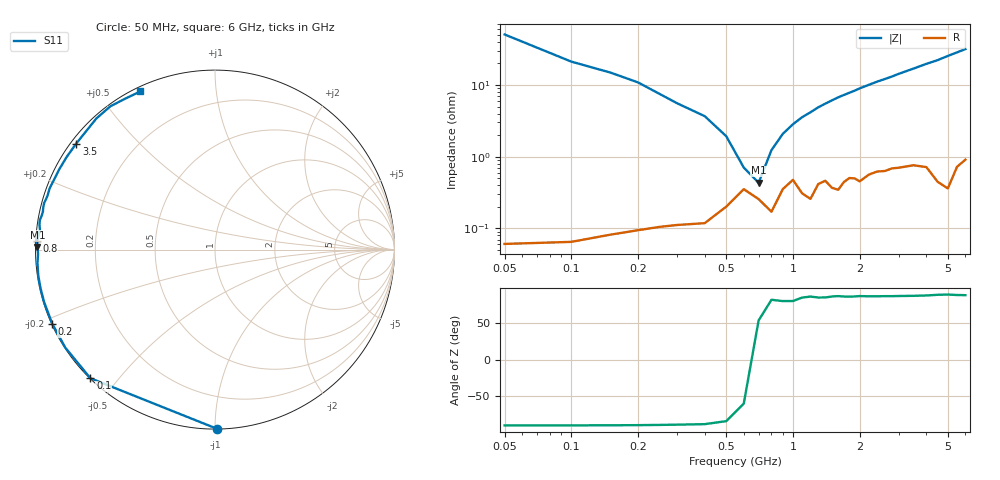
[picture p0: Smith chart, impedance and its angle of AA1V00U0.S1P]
! Infineon Technologies  Discrete & RF Semiconductors
! BBY66-02W
! Si Tuning Diode in SCD-80
! VR = 1 V
! S-Parameters:  June  2000
# GHz  S  MA  R  50
!  f  S11
! GHz  MAG  ANG
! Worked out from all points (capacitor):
!   34 points, 50 MHz to 6 GHz, reference 50 ohm
!   read as one part to ground: C = 67.5 pF near 50 MHz
!   lowest |Z| = 433 mohm at 700 MHz (marker M1)
!   series resonance near 663.6 MHz, so ESL is about 850 pH
!   S11 on the Smith chart (normalised r, x): 50 MHz: 0.00, -1.01; 100 MHz: 0.00, -0.42; 200 MHz: 0.00, -0.22; 800 MHz: 0.00, +0.02; 3.5 GHz: 0.02, +0.34; 6 GHz: 0.02, +0.63
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0.05  0.9988 -89.3
0.1  0.9978 -134.1
0.15  0.997 -146.8
0.2  0.9964 -155.5
0.25  0.9959 -162.9
0.3  0.9956 -167.3
0.4  0.9953 -171.6
0.5  0.992 -175.6
0.6  0.986 -178.6
0.7  0.9898 179.2
0.8  0.9932 177.2
1  0.9812 173.6
1.1  0.9878 171.9
1.2  0.9898 170.5
1.3  0.9837 168.9
1.4  0.9819 167.5
1.6  0.9865 164.7
1.9  0.9808 161.1
2  0.9826 159.7
2.4  0.9766 154.9
2.8  0.9746 150.6
3  0.9744 148.1
3.5  0.9731 142.6
4  0.9755 137.0
4.5  0.9852 132.1
5  0.9886 126.1
5.5  0.9784 120.7
6  0.9744 115.3
